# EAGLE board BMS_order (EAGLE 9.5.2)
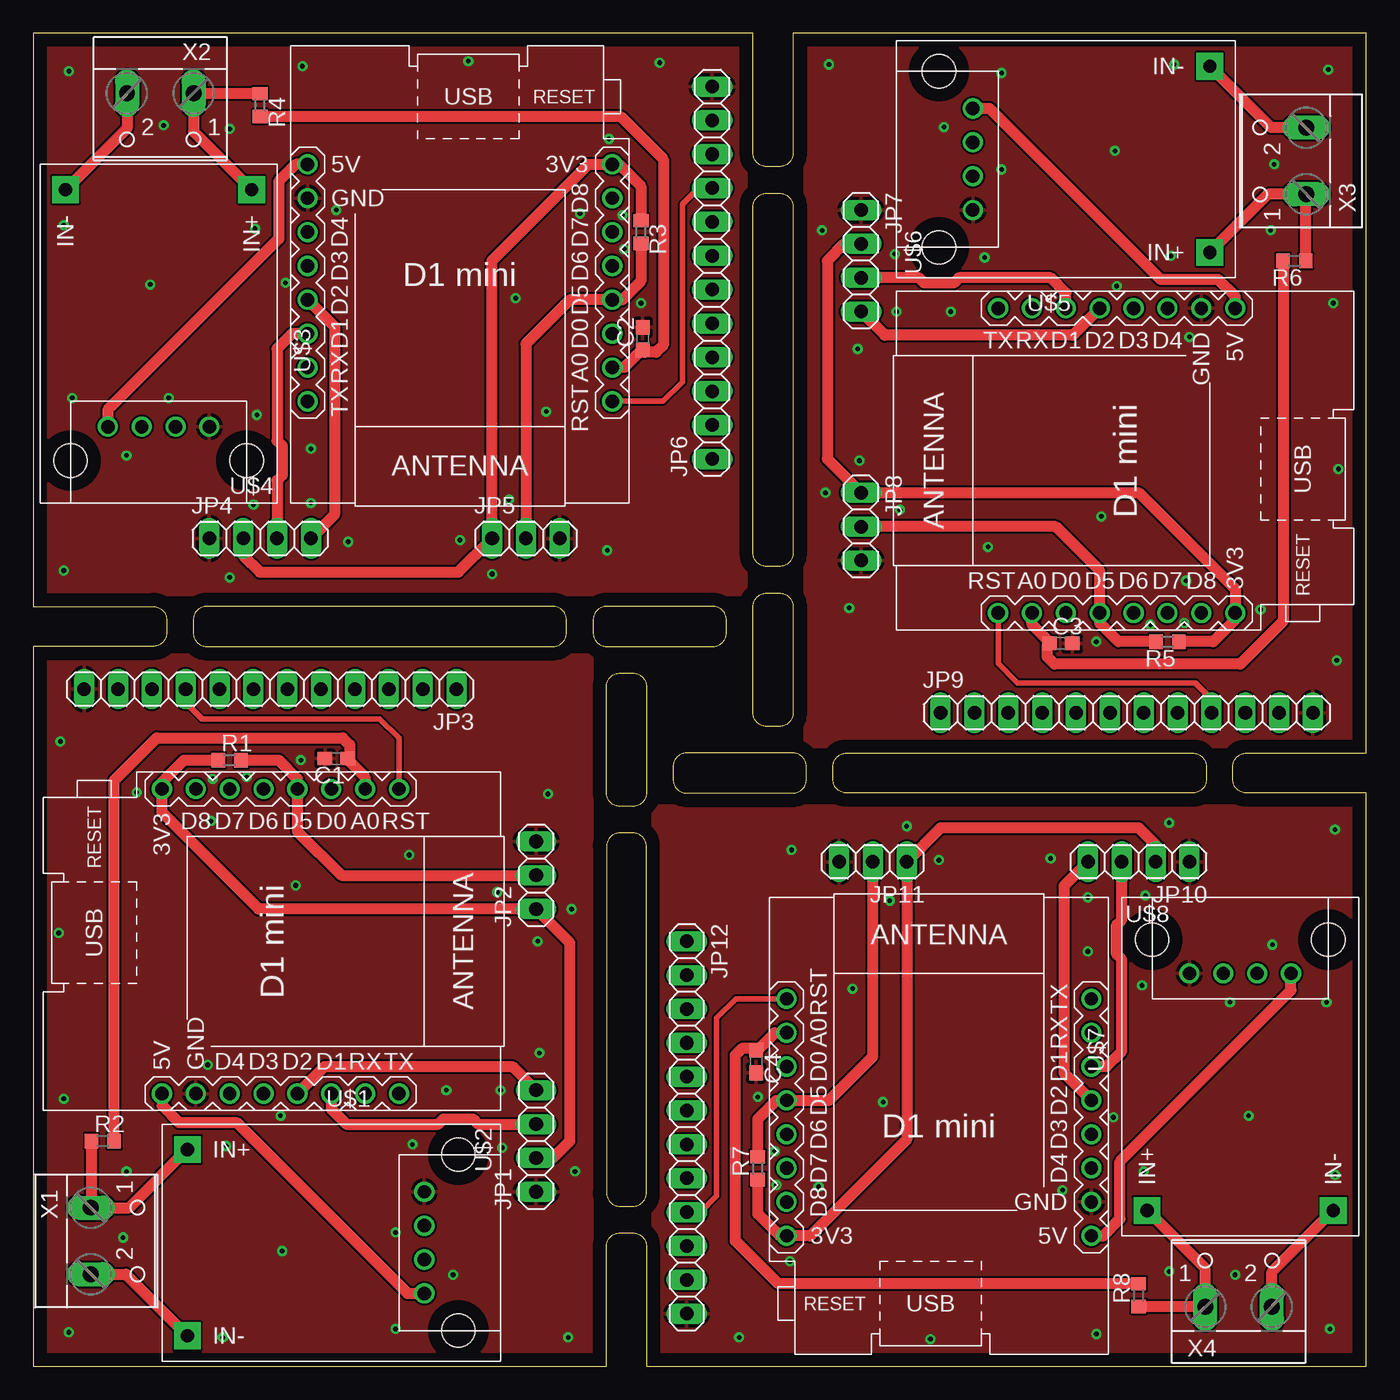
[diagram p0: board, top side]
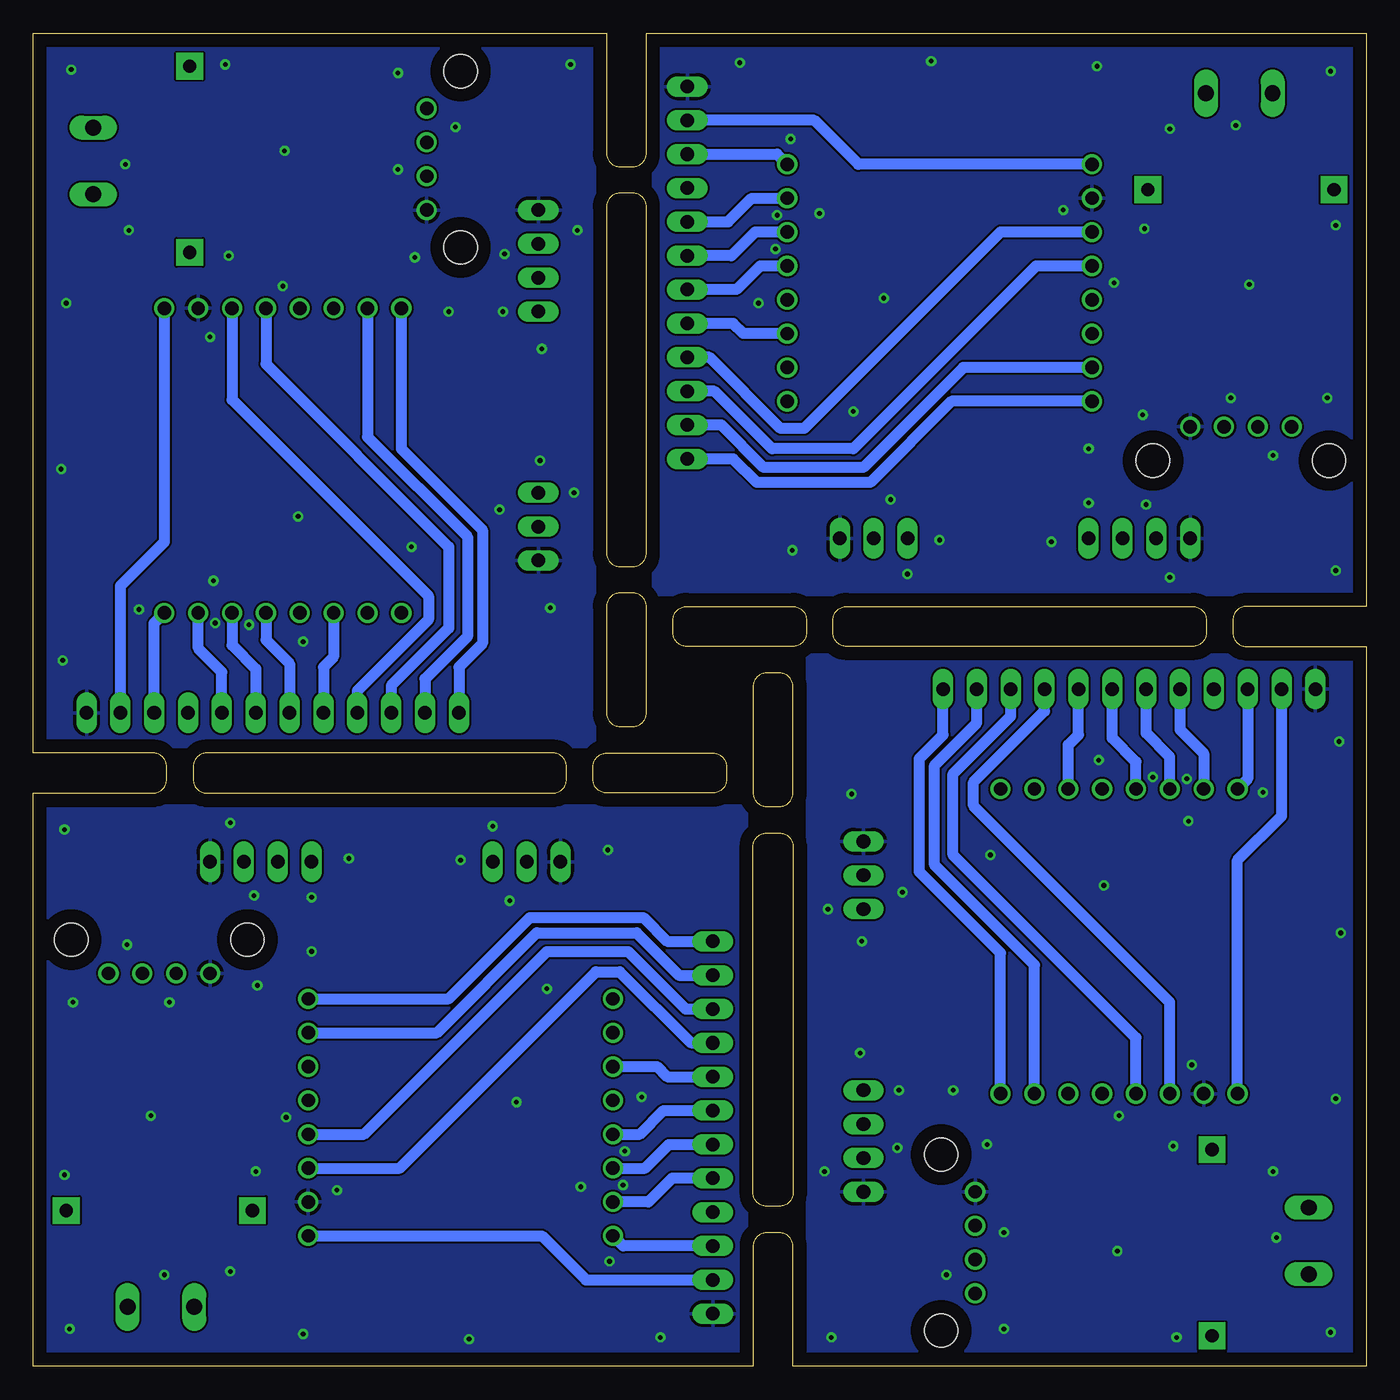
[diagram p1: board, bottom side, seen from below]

Size 100 x 100 mm. Coordinates in mm from the lower left corner, seen from the top.
Outline: 92 segments
Copper layers (1*16): Top 0.035mm / dielectric 0.15mm / Bottom 0.035mm
Design rules "default": minimum track width 6mil, minimum drill 0.35mm, track to track 6mil, track to pad 6mil, pad to pad 6mil, via to via 6mil, smd to smd 6mil, copper to edge 40mil, drill to drill 6mil, minimum pad ring 10mil, minimum via ring 8mil, stop-mask expansion 4mil, vias tented up to drill 0mil, thermal gap 10mil

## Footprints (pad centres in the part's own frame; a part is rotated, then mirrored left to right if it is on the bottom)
C0603 = smd 1.1 x 1: 1 -0.85,0; 2 0.85,0
1X04 = drill 1.016 long: 1 -3.81,0; 2 -1.27,0; 3 1.27,0; 4 3.81,0
1X03 = drill 1.016 long: 1 -2.54,0; 2 0,0; 3 2.54,0
1X12 = drill 1.016 long: 1 -13.97,0; 2 -11.43,0; 3 -8.89,0; 4 -6.35,0; 5 -3.81,0; 6 -1.27,0; 7 1.27,0; 8 3.81,0; 9 6.35,0; 10 8.89,0; 11 11.43,0; 12 13.97,0
R0603 = smd 1 x 1.1: 1 -0.85,0; 2 0.85,0
DC-DC-STEP-UP-5V = drill 1: 5V 6.985,-3.81; D+ 6.985,1.27; D- 6.985,-1.27; GND 6.985,3.81 | drill 1 pad 2 square: IN+ -10.795,6.985; IN- -10.795,-6.985 | hole 2.5: 9.525,6.604; 9.525,-6.604
WEMOS-D1-MINI = drill 1: JP1.1 -11.43,9.525; JP1.2 -11.43,6.985; JP1.3 -11.43,4.445; JP1.4 -11.43,1.905; JP1.5 -11.43,-0.635; JP1.6 -11.43,-3.175; JP1.7 -11.43,-5.715; JP1.8 -11.43,-8.255; JP2.1 11.43,9.525; JP2.2 11.43,6.985; JP2.3 11.43,4.445; JP2.4 11.43,1.905; JP2.5 11.43,-0.635; JP2.6 11.43,-3.175; JP2.7 11.43,-5.715; JP2.8 11.43,-8.255
W237-102 = drill 1.194 long: 1 -2.5,-1.27; 2 2.5,-1.27

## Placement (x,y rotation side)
C1  100n  [C0603]  22.73,45.59 180 top
C2  100n  [C0603]  45.72,77.09 90 top
C3  100n  [C0603]  77.09,54.23 0 top
C4  100n  [C0603]  54.23,22.86 270 top
JP1  [1X04]  37.72,16.89 90 top
JP2  [1X03]  37.72,36.83 90 top
JP3  [1X12]  17.78,50.8 180 top
JP4  [1X04]  17.02,62.1 0 top
JP5  [1X03]  36.96,62.1 0 top
JP6  [1X12]  50.93,82.04 90 top
JP7  [1X04]  62.1,82.93 270 top
JP8  [1X03]  62.1,62.99 270 top
JP9  [1X12]  82.04,49.02 0 top
JP10  [1X04]  82.93,37.85 180 top
JP11  [1X03]  62.99,37.85 180 top
JP12  [1X12]  49.02,17.91 270 top
R1  4k7  [R0603]  14.73,45.47 0 top
R2  100k  [R0603]  5.21,16.89 0 top
R3  4k7  [R0603]  45.59,85.09 270 top
R4  100k  [R0603]  17.02,94.61 270 top
R5  4k7  [R0603]  85.09,54.36 180 top
R6  100k  [R0603]  94.61,82.93 180 top
R7  4k7  [R0603]  54.36,14.86 90 top
R8  100k  [R0603]  82.93,5.33 90 top
U$1  DC-DC-STEP-UP-5V  [DC-DC-STEP-UP-5V]  22.35,9.27 0 top
U$2  WEMOS-D1-MINI  [WEMOS-D1-MINI]  17.91,31.88 270 top
U$3  DC-DC-STEP-UP-5V  [DC-DC-STEP-UP-5V]  9.4,77.47 270 top
U$4  WEMOS-D1-MINI  [WEMOS-D1-MINI]  32,81.92 180 top
U$5  DC-DC-STEP-UP-5V  [DC-DC-STEP-UP-5V]  77.47,90.55 180 top
U$6  WEMOS-D1-MINI  [WEMOS-D1-MINI]  81.92,67.94 90 top
U$7  DC-DC-STEP-UP-5V  [DC-DC-STEP-UP-5V]  90.55,22.48 90 top
U$8  WEMOS-D1-MINI  [WEMOS-D1-MINI]  67.94,18.03 0 top
X1  [W237-102]  5.59,9.4 270 top
X2  [W237-102]  9.53,94.23 180 top
X3  [W237-102]  94.23,90.42 90 top
X4  [W237-102]  90.42,5.71 0 top

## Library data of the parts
C1-C4 = rcl; SPICEPREFIX: C
JP1-JP12 = pinhead
R1-R8 = rcl; SPICEPREFIX: R
U$1-U$8 = diy-modules
X1-X4 = con-wago-500; MPN: 237-102; OC_FARNELL: unknown; OC_NEWARK: 70K9898

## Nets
+3V1: JP4.2 JP5.1 JP6.10 R3.1 U$4.JP1.8
+3V2: JP7.2 JP8.1 JP9.10 R5.1 U$6.JP1.8
+3V3: JP1.2 JP2.1 JP3.10 R1.1 U$2.JP1.8
+3V4: JP10.2 JP11.1 JP12.10 R7.1 U$8.JP1.8
D0: JP3.5 U$2.JP1.3
D1: JP6.3 U$4.JP2.5
D2: JP6.4 U$4.JP2.6
D3: JP3.3 U$2.JP2.5
D4: JP3.4 U$2.JP2.6
D5: JP6.5 U$4.JP1.3
D6: JP3.6 U$2.JP1.5
D7: JP3.7 U$2.JP1.6
D8: JP3.8 U$2.JP1.7
D9: JP6.6 U$4.JP1.5
D10: JP6.7 U$4.JP1.6
D11: JP6.8 U$4.JP1.7
D12: JP9.3 U$6.JP2.5
D13: JP9.4 U$6.JP2.6
D14: JP9.5 U$6.JP1.3
D15: JP9.6 U$6.JP1.5
D16: JP9.7 U$6.JP1.6
D17: JP9.8 U$6.JP1.7
D18: JP12.3 U$8.JP2.5
D19: JP12.4 U$8.JP2.6
D20: JP12.5 U$8.JP1.3
D21: JP12.6 U$8.JP1.5
D22: JP12.7 U$8.JP1.6
D23: JP12.8 U$8.JP1.7
GND: C1.2 JP1.1 JP2.3 JP3.12 U$1.GND U$2.JP2.7
GND1: C2.2 JP4.1 JP5.3 JP6.12 U$3.GND U$4.JP2.7
GND2: C3.2 JP7.1 JP8.3 JP9.12 U$5.GND U$6.JP2.7
GND3: C4.2 JP10.1 JP11.3 JP12.12 U$7.GND U$8.JP2.7
N$1: R2.1 U$1.IN+ X1.1
N$2: U$1.IN- X1.2
N$3: R4.1 U$3.IN+ X2.1
N$4: U$3.IN- X2.2
N$5: JP2.2 R1.2 U$2.JP1.4
N$6: JP5.2 R3.2 U$4.JP1.4
N$7: C1.1 R2.2 U$2.JP1.2
N$8: C2.1 R4.2 U$4.JP1.2
N$9: R6.1 U$5.IN+ X3.1
N$10: U$5.IN- X3.2
N$11: JP8.2 R5.2 U$6.JP1.4
N$12: C3.1 R6.2 U$6.JP1.2
N$13: R8.1 U$7.IN+ X4.1
N$14: U$7.IN- X4.2
N$15: JP11.2 R7.2 U$8.JP1.4
N$16: C4.1 R8.2 U$8.JP1.2
RST: JP3.9 U$2.JP1.1
RST1: JP6.9 U$4.JP1.1
RST2: JP9.9 U$6.JP1.1
RST3: JP12.9 U$8.JP1.1
RX: JP3.2 U$2.JP2.2
RX1: JP6.2 U$4.JP2.2
RX2: JP9.2 U$6.JP2.2
RX3: JP12.2 U$8.JP2.2
SCL: JP1.3 U$2.JP2.3
SCL1: JP4.3 U$4.JP2.3
SCL2: JP7.3 U$6.JP2.3
SCL3: JP10.3 U$8.JP2.3
SDA: JP1.4 U$2.JP2.4
SDA1: JP4.4 U$4.JP2.4
SDA2: JP7.4 U$6.JP2.4
SDA3: JP10.4 U$8.JP2.4
TX: JP3.1 U$2.JP2.1
TX1: JP6.1 U$4.JP2.1
TX2: JP9.1 U$6.JP2.1
TX3: JP12.1 U$8.JP2.1
VCC: JP3.11 U$1.5V U$2.JP2.8
VCC1: JP6.11 U$3.5V U$4.JP2.8
VCC2: JP9.11 U$5.5V U$6.JP2.8
VCC3: JP12.11 U$7.5V U$8.JP2.8

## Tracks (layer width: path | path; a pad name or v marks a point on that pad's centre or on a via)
+3V1
  Top 0.813: JP4.2 15.75,60.83 17.02,59.56 31.88,59.56 JP5.1 34.42,82.93 41.66,90.17 U$4.JP1.8 43.94,90.17 45.59,88.52 R3.1
  Bottom 0.813: JP6.10 44.2,90.93 U$4.JP1.8
+3V2
  Top 0.813: JP7.2 60.83,84.2 59.56,82.93 59.56,68.07 JP8.1 82.93,65.53 90.17,58.29 U$6.JP1.8 90.17,56.01 88.52,54.36 R5.1
  Bottom 0.813: JP9.10 90.93,55.75 U$6.JP1.8
+3V3
  Top 0.813: JP1.2 38.99,15.62 40.26,16.89 40.26,31.75 JP2.1 16.89,34.29 9.65,41.53 U$2.JP1.8 9.65,43.81 11.3,45.47 R1.1
  Bottom 0.813: JP3.10 8.89,44.07 U$2.JP1.8
+3V4
  Top 0.813: JP10.2 84.2,39.12 82.93,40.39 68.07,40.39 JP11.1 65.53,17.02 58.29,9.78 U$8.JP1.8 56.01,9.78 54.36,11.43 R7.1
  Bottom 0.813: JP12.10 55.75,9.02 U$8.JP1.8
D0
  Bottom 0.813: U$2.JP1.3 22.35,46.61 21.59,47.37 JP3.5
D1
  Bottom 0.813: U$4.JP2.5 24.77,82.55 38.48,68.83 44.58,68.83 48.9,73.15 JP6.3
D2
  Bottom 0.813: U$4.JP2.6 27.43,85.09 42.16,70.36 43.94,70.36 49.28,75.69 JP6.4
D3
  Bottom 0.813: U$2.JP2.5 17.27,24.64 30.99,38.35 30.99,44.45 26.67,48.77 JP3.3
D4
  Bottom 0.813: U$2.JP2.6 14.73,27.3 29.46,42.04 29.46,43.81 24.13,49.15 JP3.4
D5
  Bottom 0.813: U$4.JP1.3 46.74,77.47 47.5,78.23 JP6.5
D6
  Bottom 0.813: U$2.JP1.5 17.27,45.34 19.05,47.12 JP3.6
D7
  Bottom 0.813: U$2.JP1.6 14.73,45.72 16.51,47.5 JP3.7
D8
  Bottom 0.813: JP3.8 13.97,47.75 12.19,45.97 U$2.JP1.7
D9
  Bottom 0.813: U$4.JP1.5 45.47,82.55 47.24,80.77 JP6.6
D10
  Bottom 0.813: U$4.JP1.6 45.85,85.09 47.62,83.31 JP6.7
D11
  Bottom 0.813: JP6.8 47.88,85.85 46.1,87.63 U$4.JP1.7
D12
  Bottom 0.813: U$6.JP2.5 82.55,75.18 68.83,61.47 68.83,55.37 73.15,51.05 JP9.3
D13
  Bottom 0.813: U$6.JP2.6 85.09,72.52 70.36,57.78 70.36,56.01 75.69,50.67 JP9.4
D14
  Bottom 0.813: U$6.JP1.3 77.47,53.21 78.23,52.45 JP9.5
D15
  Bottom 0.813: U$6.JP1.5 82.55,54.48 80.77,52.7 JP9.6
D16
  Bottom 0.813: U$6.JP1.6 85.09,54.1 83.31,52.32 JP9.7
D17
  Bottom 0.813: JP9.8 85.85,52.07 87.63,53.85 U$6.JP1.7
D18
  Bottom 0.813: U$8.JP2.5 75.18,17.4 61.47,31.11 55.37,31.11 51.05,26.8 JP12.3
D19
  Bottom 0.813: U$8.JP2.6 72.52,14.86 57.78,29.59 56.01,29.59 50.67,24.26 JP12.4
D20
  Bottom 0.813: U$8.JP1.3 53.21,22.48 52.45,21.72 JP12.5
D21
  Bottom 0.813: U$8.JP1.5 54.48,17.4 52.7,19.18 JP12.6
D22
  Bottom 0.813: U$8.JP1.6 54.1,14.86 52.32,16.64 JP12.7
D23
  Bottom 0.813: JP12.8 52.07,14.1 53.85,12.32 U$8.JP1.7
GND  (via drill 0.35)
  other vias: 19.68,36.07 13.34,40.89 20.07,45.47 13.46,44.07 16,44.2 7.75,43.05 37.97,23.5 40.39,34.29 6.99,14.61 14.48,16.51 6.73,9.65 27.18,2.79 2.67,2.54 2.29,20.07 40.13,2.16 40.64,14.61 31.5,6.86 1.91,32.51 2.03,46.86 38.61,42.93 28.19,38.35 34.8,35.56 37.85,31.88 30.99,20.7 35.05,20.7 18.54,18.8 13.08,22.61 14.22,2.16 18.67,8.64 27.18,10.03 28.45,16.64 35.18,16.38
  pour Top: 0,0 0,53.34 41.91,53.34 41.91,0
  pour Bottom: 0,53.34 0,0 41.91,0 41.91,53.34
GND1  (via drill 0.35)
  other vias: 36.2,80.14 41.02,86.49 45.59,79.76 44.2,86.36 44.32,83.82 43.18,92.08 23.62,61.85 34.42,59.44 14.73,92.84 16.64,85.34 9.78,93.09 2.92,72.64 2.67,97.16 20.19,97.54 2.29,59.69 14.73,59.18 6.99,68.33 32.64,97.92 46.99,97.79 43.05,61.21 38.48,71.63 35.69,65.02 32,61.98 20.83,68.83 20.83,64.77 18.92,81.28 22.73,86.74 2.29,85.6 8.76,81.15 10.16,72.64 16.76,71.37 16.51,64.64
  pour Top: 0.13,99.82 53.47,99.82 53.47,57.91 0.13,57.91
  pour Bottom: 53.47,99.82 0.13,99.82 0.13,57.91 53.47,57.91
GND2  (via drill 0.35)
  other vias: 80.14,63.75 86.49,58.93 79.76,54.36 86.36,55.75 83.82,55.63 92.08,56.77 61.85,76.33 59.44,65.53 92.84,85.22 85.34,83.31 93.09,90.17 72.64,97.03 97.16,97.28 97.54,79.76 59.69,97.66 59.18,85.22 68.33,92.96 97.92,67.31 97.79,52.96 61.21,56.9 71.63,61.47 65.02,64.26 61.98,67.94 68.83,79.12 64.77,79.12 81.28,81.03 86.74,77.22 85.6,97.66 81.15,91.19 72.64,89.79 71.37,83.19 64.64,83.44
  pour Top: 99.82,99.82 99.82,46.48 57.91,46.48 57.91,99.82
  pour Bottom: 99.82,46.48 99.82,99.82 57.91,99.82 57.91,46.48
GND3  (via drill 0.35)
  other vias: 63.75,19.81 58.93,13.46 54.36,20.19 55.75,13.59 55.63,16.13 56.77,7.87 76.33,38.1 65.53,40.51 85.22,7.11 83.31,14.61 90.17,6.86 97.03,27.3 97.28,2.79 79.76,2.41 97.66,40.26 85.22,40.77 92.96,31.62 67.31,2.03 52.96,2.16 56.9,38.73 61.47,28.32 64.26,34.92 67.94,37.97 79.12,31.11 79.12,35.18 81.03,18.67 77.22,13.21 97.66,14.35 91.19,18.8 89.79,27.3 83.19,28.57 83.44,35.31
  pour Top: 99.82,0.13 46.48,0.13 46.48,42.04 99.82,42.04
  pour Bottom: 46.48,0.13 99.82,0.13 99.82,42.04 46.48,42.04
N$1
  Top 0.813: U$1.IN+ 7.2,11.9 X1.1 4.36,11.94 R2.1
N$2
  Top 0.813: X1.2 6.95,6.9 U$1.IN-
N$3
  Top 0.813: U$3.IN+ 12.03,92.62 X2.1 12.06,95.47 R4.1
N$4
  Top 0.813: X2.2 7.03,92.88 U$3.IN-
N$5
  Top 0.813: R1.2 18.41,45.47 19.81,44.07 U$2.JP1.4 19.81,40.13 23.11,36.83 JP2.2
N$6
  Top 0.813: R3.2 45.59,81.41 44.2,80.01 U$4.JP1.4 40.26,80.01 36.96,76.71 JP5.2
N$7
  Top 0.813: U$2.JP1.2 24.89,44.2 23.58,45.51 C1.1 23.75,45.76 23.75,46.61 23.21,47.14 9.27,47.14 6.06,43.93 R2.2
N$8
  Top 0.813: U$4.JP1.2 44.32,74.93 45.63,76.24 C2.1 45.89,76.07 46.74,76.07 47.27,76.61 47.27,90.55 44.06,93.77 R4.2
N$9
  Top 0.813: U$5.IN+ 92.62,87.92 X3.1 95.47,87.89 R6.1
N$10
  Top 0.813: X3.2 92.88,92.92 U$5.IN-
N$11
  Top 0.813: R5.2 81.41,54.36 80.01,55.75 U$6.JP1.4 80.01,59.69 76.71,62.99 JP8.2
N$12
  Top 0.813: U$6.JP1.2 74.93,55.63 76.24,54.32 C3.1 76.07,54.06 76.07,53.21 76.61,52.68 90.55,52.68 93.77,55.89 R6.2
N$13
  Top 0.813: U$7.IN+ 87.92,7.33 X4.1 87.89,4.48 R8.1
N$14
  Top 0.813: X4.2 92.92,7.07 U$7.IN-
N$15
  Top 0.813: R7.2 54.36,18.54 55.75,19.94 U$8.JP1.4 59.69,19.94 62.99,23.24 JP11.2
N$16
  Top 0.813: U$8.JP1.2 55.63,25.02 54.32,23.71 C4.1 54.06,23.88 53.21,23.88 52.68,23.34 52.68,9.4 55.89,6.18 R8.2
RST
  Top 0.406: U$2.JP1.1 27.43,47.12 25.99,48.56 12.65,48.56 11.43,49.78 JP3.9
RST1
  Top 0.406: U$4.JP1.1 47.24,72.39 48.69,73.83 48.69,87.17 49.91,88.39 JP6.9
RST2
  Top 0.406: U$6.JP1.1 72.39,52.7 73.83,51.26 87.17,51.26 88.39,50.04 JP9.9
RST3
  Top 0.406: U$8.JP1.1 52.7,27.56 51.26,26.11 51.26,12.78 50.04,11.56 JP12.9
RX
  Bottom 0.813: U$2.JP2.2 24.89,30.1 32.38,37.59 32.38,45.09 29.21,48.26 JP3.2
RX1
  Bottom 0.813: U$4.JP2.2 30.23,74.93 37.72,67.44 45.21,67.44 48.39,70.61 JP6.2
RX2
  Bottom 0.813: U$6.JP2.2 74.93,69.72 67.44,62.23 67.44,54.74 70.61,51.56 JP9.2
RX3
  Bottom 0.813: U$8.JP2.2 69.72,25.02 62.23,32.51 54.74,32.51 51.56,29.34 JP12.2
SCL
  Top 0.813: U$2.JP2.3 22.35,19.3 23.5,18.16 30.38,18.16 30.77,18.55 32.98,18.55 33.37,18.16 JP1.3
SCL1
  Top 0.813: U$4.JP2.3 19.43,77.47 18.29,76.33 18.29,69.44 18.67,69.05 18.67,66.84 18.29,66.45 JP4.3
SCL2
  Top 0.813: U$6.JP2.3 77.47,80.52 76.33,81.66 69.44,81.66 69.05,81.28 66.84,81.28 66.45,81.66 JP7.3
SCL3
  Top 0.813: U$8.JP2.3 80.52,22.48 81.66,23.62 81.66,30.51 81.28,30.9 81.28,33.11 81.66,33.5 JP10.3
SDA
  Top 0.813: U$2.JP2.4 21.84,22.48 35.94,22.48 JP1.4
SDA1
  Top 0.813: U$4.JP2.4 22.61,77.98 22.61,63.88 JP4.4
SDA2
  Top 0.813: U$6.JP2.4 77.98,77.34 63.88,77.34 JP7.4
SDA3
  Top 0.813: U$8.JP2.4 77.34,21.97 77.34,36.07 JP10.4
TX
  Bottom 0.813: U$2.JP2.1 27.43,30.99 33.53,37.08 33.53,45.59 31.75,47.37 JP3.1
TX1
  Bottom 0.813: U$4.JP2.1 31.11,72.39 37.21,66.29 45.72,66.29 47.5,68.07 JP6.1
TX2
  Bottom 0.813: U$6.JP2.1 72.39,68.83 66.29,62.74 66.29,54.23 68.07,52.45 JP9.1
TX3
  Bottom 0.813: U$8.JP2.1 68.83,27.56 62.74,33.66 54.23,33.66 52.45,31.88 JP12.1
VCC
  Top 0.813: U$2.JP2.8 9.65,19.56 10.92,18.29 15.24,18.29 28.07,5.46 U$1.5V
  Bottom 0.813: U$2.JP2.8 9.65,37.97 6.35,41.27 JP3.11
VCC1
  Top 0.813: U$4.JP2.8 19.68,90.17 18.41,88.9 18.41,84.58 5.59,71.75 U$3.5V
  Bottom 0.813: U$4.JP2.8 38.1,90.17 41.4,93.47 JP6.11
VCC2
  Top 0.813: U$6.JP2.8 90.17,80.26 88.9,81.53 84.58,81.53 71.75,94.36 U$5.5V
  Bottom 0.813: U$6.JP2.8 90.17,61.85 93.47,58.55 JP9.11
VCC3
  Top 0.813: U$8.JP2.8 80.26,9.78 81.53,11.05 81.53,15.37 94.36,28.19 U$7.5V
  Bottom 0.813: U$8.JP2.8 61.85,9.78 58.55,6.48 JP12.11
